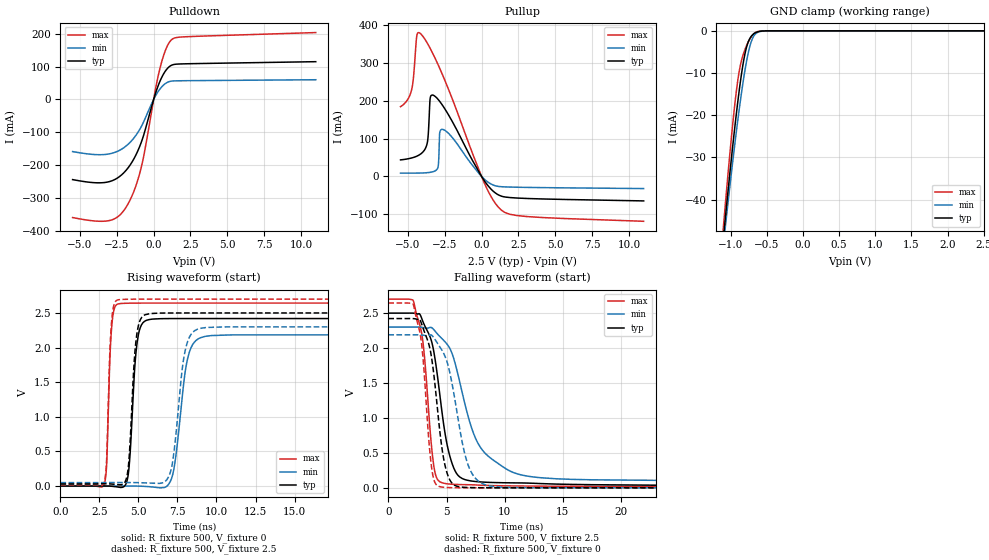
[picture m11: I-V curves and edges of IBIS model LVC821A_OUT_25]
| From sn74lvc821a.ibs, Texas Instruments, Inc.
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[Model]   LVC821A_OUT_25
Model_type  3-state
Enable   Active-Low
Vref =   0
Rref =   500
Cref =   30p
Vmeas =   1.25
| variable   typ   min   max
C_comp   6.69pF   6.01pF   7.81pF
| C_pullup   8.54pF   7.48pF   9.77pF
| C_pulldown   12.39pF   7.81pF   19.53pF
| C_tri-state   6.69pF   6.01pF   7.81pF
[Temperature Range]   40   100   -40
| Ambient temperature   25   85   -40
[Voltage range]   2.5   2.3   2.7
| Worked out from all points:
|   slope of the pulldown table from 0 to 0.375 V, typ, clamps not added: 7.52 ohm
|   slope of the pullup table from 0 to 0.375 V, typ, clamps not added: 17.6 ohm
|   GND clamp passes 1 mA (typ) near -0.70 V on its own axis
|   rising waveform, R_fixture 500, V_fixture 0: 20-80 % time 377ps typ, 668ps min, 231ps max; typ from 0 V to 2.42 V
|   falling waveform, R_fixture 500, V_fixture 2.5: 20-80 % time 1.33ns typ, 2.56ns min, 826ps max; typ from 2.5 V to 0.034 V
|   rising waveform, R_fixture 500, V_fixture 2.5: 20-80 % time 365ps typ, 624ps min, 226ps max; typ from 0.032 V to 2.5 V
|   falling waveform, R_fixture 500, V_fixture 0: 20-80 % time 1.05ns typ, 1.52ns min, 746ps max; typ from 2.42 V to 0 V
[GND Clamp]
| LVC821A_OUT_25
|   Voltage   I(typ)   I(min)   I(max)
-5.5V     -1.089A    -967.7mA   -1.248A
-1.1V     -48.78mA   -50.46mA   -46.17mA
-1.07V    -43.53mA   -45.73mA   -40.17mA
-965mV    -26.13mA   -29.91mA   -20.85mA
-925mV    -20.06mA   -24.27mA   -14.68mA
-885mV    -14.46mA   -18.92mA   -9.824mA
-830mV    -7.921mA   -12.23mA   -5.763mA
-780mV    -3.803mA   -7.105mA   -3.458mA
-720mV    -1.391mA   -2.774mA   -1.488mA
-650mV    -377.7uA   -605.1uA   -336.4uA
-445mV    -2.091uA   -3.632uA   -593.1nA
2.5V      55.16pA    1.186nA    52.88pA
[Pulldown]
| LVC821A_OUT_25
|   Voltage   I(typ)   I(min)   I(max)
-5.5V     -244.6mA   -159.1mA   -360.4mA
-2.955V   -250mA     -165.6mA   -369mA
-2.31V    -235mA     -155.1mA   -353.3mA
-1.735V   -208.7mA   -136.8mA   -318.6mA
-1.235V   -172.1mA   -111.4mA   -267.4mA
-810mV    -126.9mA   -80.28mA   -201.2mA
-555mV    -89.7mA    -55.62mA   -144.1mA
145mV     21.26mA    12.4mA     36.27mA
500mV     62.85mA    35.97mA    107.7mA
880mV     91.77mA    50.98mA    158.6mA
1.255V    105.2mA    56.25mA    183.9mA
11V       115.3mA    60.21mA    204.2mA
[Pullup]
| LVC821A_OUT_25
|   Voltage   I(typ)   I(min)   I(max)
-5.5V     43.69mA    8.685mA    184mA
-4.755V   48.65mA    8.717mA    227.4mA
-4.405V   53.28mA    8.819mA    368.6mA
-4.23V    56.77mA    8.927mA    379.3mA
-3.7V     85.97mA    9.87mA     352.9mA
-3.49V    205.6mA    10.82mA    338.1mA
-3.255V   214mA      12.91mA    320.1mA
-2.95V    203.3mA    25.54mA    294.8mA
-2.84V    198mA      115.2mA    285.2mA
-2.625V   186.2mA    124.1mA    265.9mA
1.34V     -51.98mA   -27.1mA    -88.69mA
11V       -64.59mA   -32.03mA   -118.4mA
[Ramp]
| LVC821A_OUT_25
| variable   typ   min   max
dV/dt_r   1.46/3.83E-10   1.33/6.80E-10   1.59/2.46E-10
dV/dt_f   1.48/1.34E-09   1.33/2.55E-09   1.61/8.30E-10
R_load = 500
[Rising Waveform]
| LVC821A_OUT_25
R_fixture =   500
C_fixture =   0
L_fixture =   0
V_fixture =   0
V_fixture_min = 0
V_fixture_max = 0
|   Time   V(typ)   V(min)   V(max)
0s        457.6pV    716.6pV    260.5pV
2.84ns    1.207mV    86.45uV    48.41mV
3.27ns    -2.397mV   841.8uV    2.262V
3.68ns    -13.09mV   1.021mV    2.63V
4.34ns    159.1mV    1.025mV    2.641V
4.885ns   2.022V     39.94uV    2.643V
5.505ns   2.393V     -5.481mV   2.643V
7.12ns    2.419V     109.6mV    2.643V
8.985ns   2.42V      2.144V     2.643V
29.99ns   2.42V      2.185V     2.643V
[Falling Waveform]
| LVC821A_OUT_25
R_fixture =   500
C_fixture =   0
L_fixture =   0
V_fixture =   2.5
V_fixture_min = 2.3
V_fixture_max = 2.7
|   Time   V(typ)   V(min)   V(max)
0s        2.5V       2.3V       2.7V
2.18ns    2.499V     2.3V       2.66V
2.97ns    2.38V      2.294V     2.088V
3.68ns    2.116V     2.295V     649.2mV
4.47ns    1.272V     2.158V     83.06mV
5.13ns    557.5mV    2.037V     56.59mV
5.955ns   185.8mV    1.642V     48.11mV
7.7ns     87.68mV    640mV      39.91mV
10.46ns   71.98mV    239.9mV    28.02mV
29.99ns   34.34mV    80.19mV    20.52mV
[Rising Waveform]
| LVC821A_OUT_25
R_fixture =   500
C_fixture =   0
L_fixture =   0
V_fixture =   2.5
V_fixture_min = 2.3
V_fixture_max = 2.7
|   Time   V(typ)   V(min)   V(max)
0s        32.16mV    50.44mV    20.39mV
2.825ns   33.19mV    50.52mV    68.2mV
3.23ns    30.44mV    51.19mV    2.225V
3.62ns    22.84mV    51.26mV    2.685V
4.295ns   184.4mV    51.09mV    2.698V
4.825ns   2.066V     50.27mV    2.699V
5.42ns    2.474V     46.44mV    2.7V
7.03ns    2.5V       188.8mV    2.7V
8.775ns   2.5V       2.265V     2.7V
29.99ns   2.5V       2.3V       2.7V
[Falling Waveform]
| LVC821A_OUT_25
R_fixture =   500
C_fixture =   0
L_fixture =   0
V_fixture =   0
V_fixture_min = 0
V_fixture_max = 0
|   Time   V(typ)   V(min)   V(max)
0s        2.422V     2.19V      2.644V
2.185ns   2.421V     2.19V      2.601V
2.88ns    2.336V     2.187V     2.026V
3.52ns    2.03V      2.186V     601.4mV
4.27ns    1.05V      2.057V     26.93mV
4.765ns   408.2mV    1.921V     8.863mV
5.335ns   98.64mV    1.609V     3.822mV
6.705ns   6.375mV    405.2mV    1.059mV
8.095ns   2.044mV    60.15mV    1.091mV
29.99ns   203.4uV    730.5uV    47.62uV
